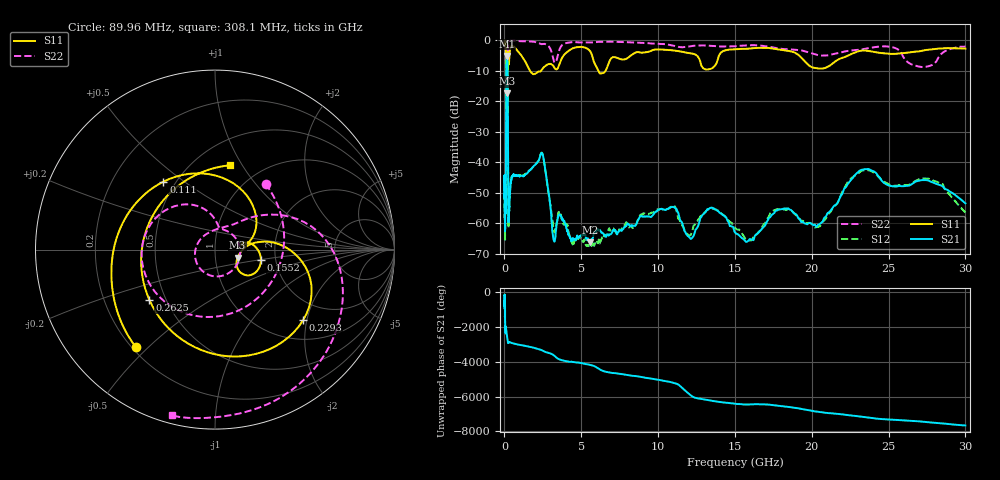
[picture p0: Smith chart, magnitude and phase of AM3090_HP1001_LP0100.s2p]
! Date/Time: Thu, Feb 28, 2019 2:03 PM
! Network Analyzer: Agilent Technologies E8364B Rev: A.07.50.67
! Sweep from 0.010 to 30.000 GHz, 1601 Points, Sweep Type: LOG
! Power Supply: 5.023 V, 0.002 A
# Hz S DB R 50
!freq MagS11 AngS11 MagS21 AngS21 MagS12 AngS12 MagS22 AngS22
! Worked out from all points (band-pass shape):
!   1601 points, 10 MHz to 30 GHz, reference 50 ohm
!   highest |S21| = -5.22 dB at 156 MHz (marker M1); lowest = -66.2 dB at 5.584 GHz (marker M2)
!   |S21| within 3 dB of the highest: 123.7 MHz to 199.7 MHz (75.99 MHz wide, 47 % of centre)
!   lowest |S11| = -17.5 dB at 189.6 MHz (marker M3), VSWR 1.31, Z = 64 - j5.95 ohm
!   |S11| at or under -10 dB: 120.6 MHz to 209.1 MHz (88.52 MHz wide, 53.7 % of centre); 1.648 GHz to 2.391 GHz (742.7 MHz wide, 36.8 % of centre); 6.102 GHz to 6.59 GHz (488.5 MHz wide, 7.7 % of centre)
!   |S22| runs from -20.1 to -0.2 dB; largest |S21 - S12| = 0.0097
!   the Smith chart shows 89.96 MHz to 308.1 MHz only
!   S11 on the Smith chart (normalised r, x): 89.96 MHz: 0.21, -0.46; 111 MHz: 0.43, +0.42; 155.2 MHz: 1.67, -0.21; 229.3 MHz: 1.46, -1.90; 262.5 MHz: 0.41, -0.29; 308.1 MHz: 0.73, +0.88
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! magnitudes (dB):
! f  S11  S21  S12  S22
! 10 MHz  -0.2  -44.2  -49.1  -0.5
! 38.04 MHz  -0.5  -60.1  -60.4  -1.3
! 89.96 MHz  -3.1  -50.2  -49.3  -6.7
! 111 MHz  -6.5  -19.3  -19.4  -7.7
! 144.7 MHz  -13.3  -5.3  -5.3  -17.7
! 155.2 MHz  -11.6  -5.2  -5.2  -16.6
! 156 MHz  -11.6  -5.2  -5.2  -16.6
! 189.6 MHz  -17.5  -6.5  -6.5  -19.9
! 209.6 MHz  -9.8  -12.9  -12.9  -11.8
! 229.3 MHz  -4.0  -40.6  -40.1  -2.8
! 262.5 MHz  -6.7  -59.2  -61.2  -0.8
! 308.1 MHz  -6.4  -55.9  -54.8  -0.4
! 550.5 MHz  -2.0  -44.4  -44.5  -0.2
! 2.084 GHz  -10.8  -40.4  -40.4  -0.8
! 2.52 GHz  -9.2  -38.1  -38.2  -1.3
! 3.22 GHz  -8.8  -65.7  -62.7  -7.0
! 5.584 GHz  -3.7  -66.2  -66.4  -0.8
! 7.926 GHz  -6.2  -61.0  -59.7  -0.7
! 15.89 GHz  -2.8  -65.7  -65.6  -1.7
! 20.41 GHz  -9.3  -60.5  -61.2  -5.0
! 23.48 GHz  -3.5  -42.3  -42.6  -2.9
! 30 GHz  -2.8  -53.5  -56.6  -2.2
